FUNCTION "Gest Semi / Automatico" : VOID
TITLE =GESTIONE AUTOMATICO 2nd CONTROLLO CORTI
VERSION : 0.1

BEGIN
NETWORK
TITLE =Start ciclo automatico
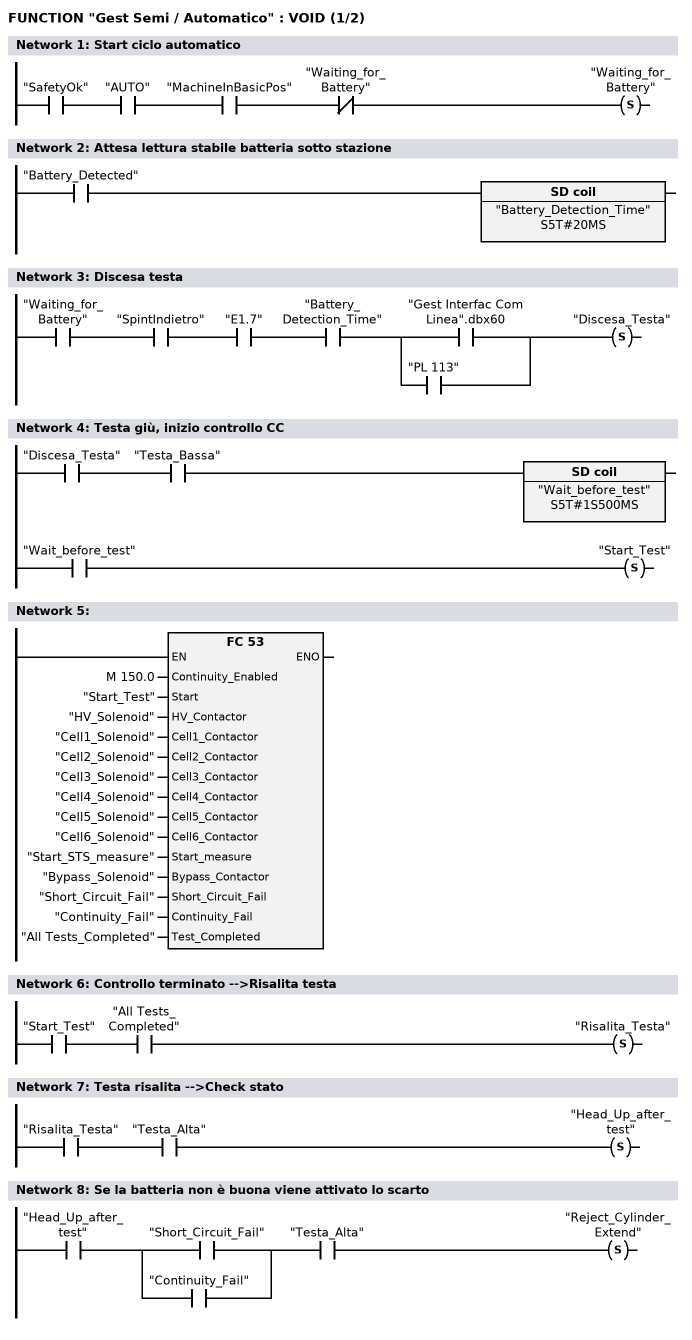
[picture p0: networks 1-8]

      U     "SafetyOk";
      U     "AUTO";
      U     "MachineInBasicPos";
      UN    "Waiting_for_Battery";
      S     "Waiting_for_Battery";
NETWORK
TITLE =Attesa lettura stabile batteria sotto stazione

      U     "Battery_Detected";
      L     S5T#20MS;
      SE    "Battery_Detection_Time";
      NOP   0;
      NOP   0;
      NOP   0;
      NOP   0;
NETWORK
TITLE =Discesa testa

      U     "Waiting_for_Battery";
      U     "SpintIndietro";
      U     "E1.7";
      U     "Battery_Detection_Time";
      U(    ;
      O     "Gest Interfac Com Linea".dbx60;
      O     "PL 113";
      )     ;
      S     "Discesa_Testa";
NETWORK
TITLE =Testa giù, inizio controllo CC

      U     "Discesa_Testa";
      U     "Testa_Bassa";
      L     S5T#1S500MS;
      SE    "Wait_before_test";
      NOP   0;
      NOP   0;
      NOP   0;
      U     "Wait_before_test";
      S     "Start_Test";
NETWORK
TITLE =

      CALL FC    53 (
           Continuity_Enabled       := M    150.0,
           Start                    := "Start_Test",
           HV_Contactor             := "HV_Solenoid",
           Cell1_Contactor          := "Cell1_Solenoid",
           Cell2_Contactor          := "Cell2_Solenoid",
           Cell3_Contactor          := "Cell3_Solenoid",
           Cell4_Contactor          := "Cell4_Solenoid",
           Cell5_Contactor          := "Cell5_Solenoid",
           Cell6_Contactor          := "Cell6_Solenoid",
           Start_measure            := "Start_STS_measure",
           Bypass_Contactor         := "Bypass_Solenoid",
           Short_Circuit_Fail       := "Short_Circuit_Fail",
           Continuity_Fail          := "Continuity_Fail",
           Test_Completed           := "All Tests_Completed");



NETWORK
TITLE =Controllo terminato -->Risalita testa

      U     "Start_Test";
      U     "All Tests_Completed";
      S     "Risalita_Testa";
NETWORK
TITLE =Testa risalita -->Check stato

      U     "Risalita_Testa";
      U     "Testa_Alta";
      S     "Head_Up_after_test";
NETWORK
TITLE =Se la batteria non è buona viene attivato lo scarto

      U     "Head_Up_after_test";
      U(    ;
      O     "Short_Circuit_Fail";
      O     "Continuity_Fail";
      )     ;
      U     "Testa_Alta";
      S     "Reject_Cylinder_Extend";
NETWORK
TITLE =Spintore torna indietro verso posizione base
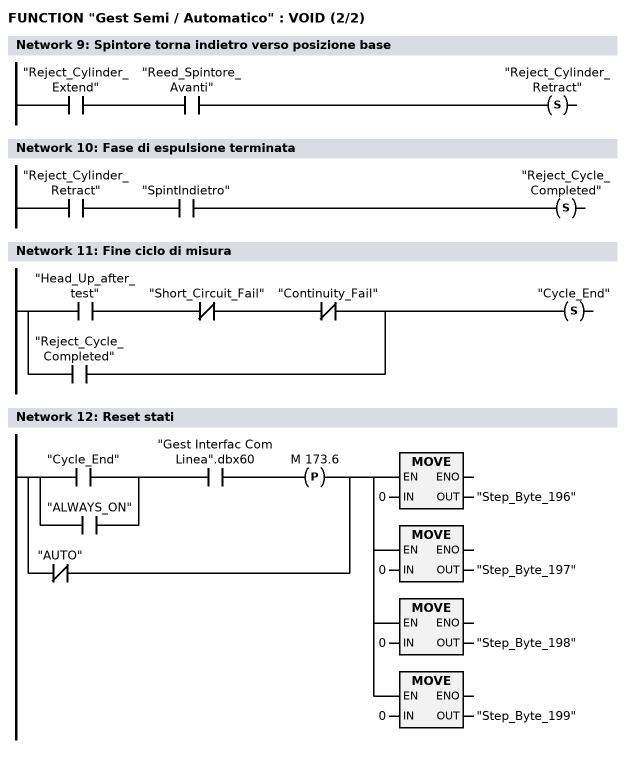
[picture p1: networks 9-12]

      U     "Reject_Cylinder_Extend";
      U     "Reed_Spintore_Avanti";
      S     "Reject_Cylinder_Retract";
NETWORK
TITLE =Fase di espulsione terminata

      U     "Reject_Cylinder_Retract";
      U     "SpintIndietro";
      S     "Reject_Cycle_Completed";
NETWORK
TITLE =Fine ciclo di misura

      U     "Head_Up_after_test";
      UN    "Short_Circuit_Fail";
      UN    "Continuity_Fail";
      O     "Reject_Cycle_Completed";
      S     "Cycle_End";
NETWORK
TITLE =Reset stati

      U(    ;
      O     "Cycle_End";
      O     "ALWAYS_ON";
      )     ;
      U     "Gest Interfac Com Linea".dbx60;
      FP    M    173.6;
      ON    "AUTO";
      =     L      0.0;
      U     L      0.0;
      SPBNB _001;
      L     0;
      T     "Step_Byte_196";
_001: NOP   0;
      U     L      0.0;
      SPBNB _002;
      L     0;
      T     "Step_Byte_197";
_002: NOP   0;
      U     L      0.0;
      SPBNB _003;
      L     0;
      T     "Step_Byte_198";
_003: NOP   0;
      U     L      0.0;
      SPBNB _004;
      L     0;
      T     "Step_Byte_199";
_004: NOP   0;
END_FUNCTION

